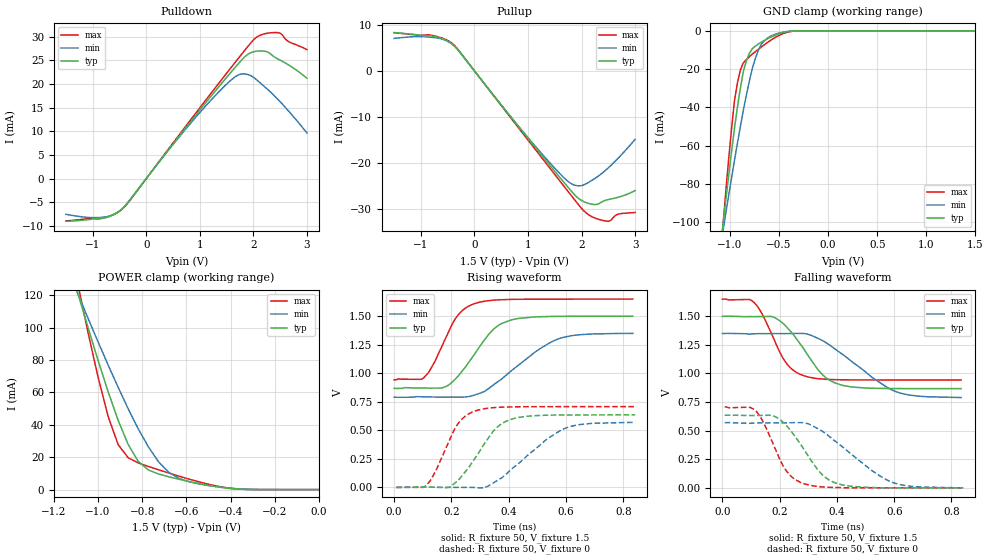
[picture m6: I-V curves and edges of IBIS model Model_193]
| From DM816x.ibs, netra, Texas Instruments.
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| Model based on original model for BSHTLTCSCDDVGPBFZ
|   Sub model FAST_6MA_10PER_P_1P5
[model]   Model_193
|[Description]  1.5V-3-STATE-X-FAST, 6MA, +-10%
|[Input Load]
|[Output Drive] FAST, 6MA
|Voltage   1.5V
|Mode   3-STATE
Model_type   3-state
Polarity   Non-Inverting
Enable   Active-Low
Cref =  15.0000pF
Rref =  100.0000M
Vref =  0V
Vmeas =  0.75
C_comp   1.5249p   1.4275p   1.6205p
[Model Spec]
[Temperature Range]   25   125   -40
[Voltage Range]   1.5   1.35   1.65
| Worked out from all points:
|   slope of the pulldown table from 0 to 0.225 V, typ, clamps not added: 67.5 ohm
|   slope of the pullup table from 0 to 0.225 V, typ, clamps not added: 67.5 ohm
|   GND clamp passes 1 mA (typ) near -0.47 V on its own axis
|   POWER clamp passes 1 mA (typ) near -0.42 V on its own axis
|   rising waveform, R_fixture 50, V_fixture 1.5: 20-80 % time 112ps typ, 175ps min, 84.6ps max; typ from 0.868 V to 1.5 V
|   rising waveform, R_fixture 50, V_fixture 0: 20-80 % time 107ps typ, 164ps min, 81ps max; typ from 0 V to 0.636 V
|   falling waveform, R_fixture 50, V_fixture 1.5: 20-80 % time 112ps typ, 181ps min, 83.8ps max; typ from 1.5 V to 0.867 V
|   falling waveform, R_fixture 50, V_fixture 0: 20-80 % time 108ps typ, 174ps min, 81.2ps max; typ from 0.635 V to 0 V
[POWER_clamp]
-1.5V     321.6mA    260.6mA    415.8mA
-1.091V   121.1mA    120.8mA    126.6mA
-1.076V   114.1mA    115.8mA    116.8mA
-1V       79.88mA    91.3mA     69.56mA
-954.5mV  60.58mA    77.05mA    45.34mA
-909.1mV  42.84mA    63.2mA     27.8mA
-818.2mV  17.47mA    37.6mA     16.51mA
-772.7mV  12.19mA    26.53mA    14.33mA
-681.8mV  7.985mA    10.89mA    10.33mA
-590.9mV  5.092mA    4.952mA    6.596mA
-363.6mV  298.9uA    465.6uA    298.1uA
0V        1.518nA    23.05nA    396.5pA
[Pulldown]
-1.5V     -9.02mA    -7.54mA    -8.95mA
-772.7mV  -8.299mA   -8.105mA   -8.235mA
-590.9mV  -7.513mA   -7.517mA   -7.478mA
-409.1mV  -5.951mA   -5.915mA   -6.017mA
954.5mV   13.88mA    13.38mA    14.3mA
1.455V    20.79mA    19.48mA    21.63mA
1.727V    24.39mA    21.97mA    25.55mA
2V        26.82mA    21.46mA    29.32mA
2.318V    26.42mA    18.34mA    30.84mA
2.5V      25.05mA    16.26mA    30.79mA
2.636V    24.2mA     14.57mA    29.14mA
3V        21.24mA    9.67mA     27.28mA
[Pullup]
-1.5V     8.32mA     7.05mA     8.28mA
-818.2mV  7.591mA    7.315mA    7.769mA
-409.1mV  5.809mA    5.727mA    5.921mA
1.227V    -17.92mA   -17.56mA   -18.4mA
1.682V    -24.33mA   -23.3mA    -25.16mA
1.864V    -26.79mA   -24.75mA   -27.86mA
2V        -28.11mA   -24.88mA   -29.82mA
2.182V    -28.88mA   -23.81mA   -31.56mA
2.409V    -28.22mA   -21.94mA   -32.46mA
2.545V    -27.79mA   -20.51mA   -32.42mA
2.682V    -27.41mA   -18.93mA   -31.08mA
3V        -25.95mA   -14.85mA   -30.69mA
[GND_clamp]
-1.5V     -310mA     -250.5mA   -402.4mA
-1.076V   -103.5mA   -106.1mA   -105.2mA
-1.045V   -89.74mA   -96.32mA   -85.93mA
-954.5mV  -51.19mA   -67.85mA   -36.85mA
-924.2mV  -40.06mA   -58.84mA   -27.27mA
-863.6mV  -21.23mA   -41.55mA   -16.73mA
-833.3mV  -15.79mA   -33.74mA   -15.03mA
-772.7mV  -9.342mA   -19.74mA   -12.19mA
-712.1mV  -6.927mA   -10.35mA   -9.702mA
-621.2mV  -4.26mA    -3.894mA   -6.224mA
-409.1mV  -336.9uA   -288.9uA   -618.6uA
1.5V      1.518nA    2.298uA    269.6pA
[Ramp]
dV/dt_f   0.50628/0.16963526n   0.448464/0.25774176n   0.565872/0.13154817n
dV/dt_r 0.51054312/0.16159714n 0.45989816/0.23732455n 0.56646706/0.12704445n
R_load = 50
[Rising Waveform]
R_fixture = 50
V_fixture = 1.5
V_fixture_min = 1.35
V_fixture_max = 1.65
0s        867.9mV    790.4mV    943mV
103.6ps   870.6mV    792.9mV    961.1mV
140ps     870mV      792.2mV    1.093V
190.2ps   897.3mV    791.9mV    1.363V
230ps     996mV      791.2mV    1.53V
280.4ps   1.165V     809.1mV    1.61V
344.3ps   1.38V      893.5mV    1.64V
410.8ps   1.469V     1.025V     1.648V
574.5ps   1.499V     1.302V     1.65V
833.3ps   1.5V       1.35V      1.65V
[Rising Waveform]
R_fixture = 50
V_fixture = 0
V_fixture_min = 0
V_fixture_max = 0
8.21ps    0V         0V         0V
110.3ps   3.137mV    2.88mV     13.94mV
146.1ps   2.167mV    2.314mV    147.8mV
196ps     7.232mV    0V         428.5mV
237.3ps   102.3mV    0V         599.7mV
290.1ps   283.2mV    -3.633mV   675.6mV
359.8ps   527.5mV    59.19mV    700.9mV
423.9ps   607.4mV    188.3mV    706mV
602.1ps   634.6mV    522.2mV    707.8mV
841.5ps   635.6mV    570.2mV    707.9mV
[Falling Waveform]
R_fixture = 50
V_fixture = 1.5
V_fixture_min = 1.35
V_fixture_max = 1.65
0s        1.499V     1.349V     1.649V
112.2ps   1.496V     1.347V     1.616V
140.9ps   1.497V     1.347V     1.511V
173.1ps   1.496V     1.348V     1.339V
215ps     1.43V      1.348V     1.121V
280.3ps   1.229V     1.349V     983.1mV
348.9ps   991mV      1.288V     951.4mV
419.9ps   895.7mV    1.166V     944.4mV
604.2ps   867.8mV    842.9mV    942.8mV
833.3ps   867.2mV    789.5mV    942.7mV
[Falling Waveform]
R_fixture = 50
V_fixture = 0
V_fixture_min = 0
V_fixture_max = 0
8.21ps    634.6mV    569.7mV    707.3mV
114.3ps   631.9mV    566.7mV    679.7mV
136.5ps   633mV      567.5mV    604.6mV
174.4ps   631.1mV    568.5mV    401.6mV
219.8ps   554mV      568.1mV    162mV
288.8ps   321.1mV    566.8mV    32.89mV
351.8ps   107.9mV    490.3mV    7.931mV
418.6ps   26.1mV     360.4mV    0V
595.6ps   0V         46.5mV     0V
841.5ps   0V         0V         0V
